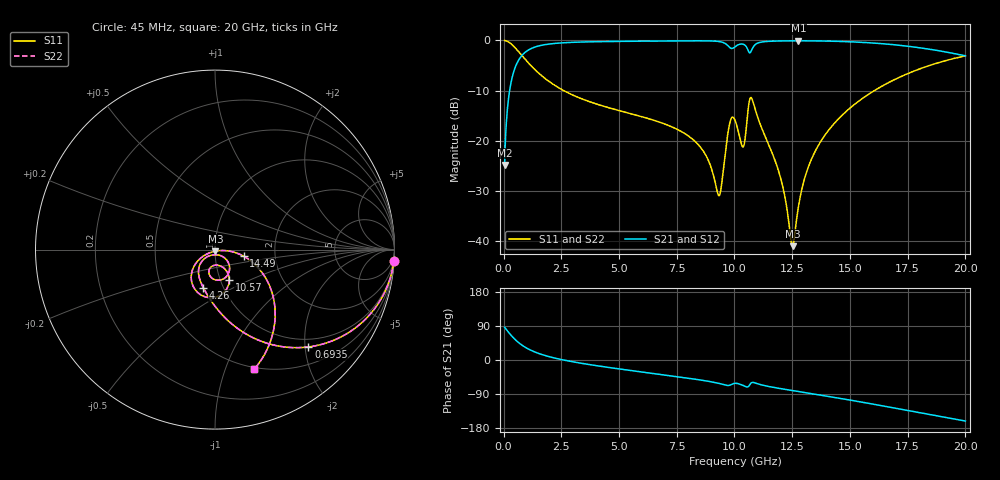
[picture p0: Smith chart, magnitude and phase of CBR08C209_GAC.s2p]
! S-parameter model data by Modelithics Inc.  support@modelithics.com 813-866-6335  Tampa FL USA
! S-Parameter data specifications:
! Substrate: 20-mil Rogers 4350B, substrate thickness, H=0.508mm, Dielectric constant, Er=3.75
! PCB Mounting Pad Footprint: Pad width, PadW=1.45mm , Pad length, PadL=1mm , Pad gap, PadG (edge-to-edge)=0.6mm , Reference planes=2.6mm apart
#  GHz  S  MA  R 50
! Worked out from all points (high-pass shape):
!   801 points, 45 MHz to 20 GHz, reference 50 ohm
!   highest |S21| = -0.09 dB at 12.77 GHz (marker M1); lowest = -24.8 dB at 45 MHz (marker M2)
!   |S21| within 3 dB of the highest: 779.9 MHz to end of sweep
!   lowest |S11| = -41.0 dB at 12.52 GHz (marker M3), VSWR 1.02, Z = 50.2 - j0.871 ohm
!   |S11| at or under -10 dB: 2.604 GHz to 16.06 GHz (13.46 GHz wide, 144 % of centre)
!   |S22| runs from -41.0 to 0.0 dB; largest |S21 - S12| = 0
!   S11 on the Smith chart (normalised r, x): 45 MHz: 1, -32; 693.5 MHz: 0.83, -2.07; 4.26 GHz: 0.81, -0.36; 10.57 GHz: 1.10, -0.38; 14.49 GHz: 1.38, -0.10; 20 GHz: 0.48, -1.26
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0.045  0.9983 -3.6  0.0573 86.4  0.0573 86.4  0.9983 -3.6
0.294438  0.9362 -22.7  0.3511 67.3  0.3511 67.3  0.9362 -22.7
0.693538  0.7514 -46.2  0.6591 43.7  0.6591 43.7  0.7514 -46.2
1.6414  0.4463 -75.1  0.8936 14.8  0.8936 14.8  0.4463 -75.1
3.387462  0.2616 -98.5  0.9634 -8.8  0.9634 -8.8  0.2616 -98.5
4.260494  0.2234 -106.7  0.9727 -17.1  0.9727 -17.1  0.2234 -106.7
6.704981  0.1547 -126.6  0.985 -37.4  0.985 -37.4  0.1547 -126.6
8.475988  0.08917 -139.0  0.9899 -52.3  0.9899 -52.3  0.08917 -139.0
9.324075  0.02834 -91.8  0.9744 -61.8  0.9744 -61.8  0.02834 -91.8
9.773062  0.1416 -55.4  0.8598 -66.8  0.8598 -66.8  0.1416 -55.4
10.0225  0.1601 -96.0  0.863 -61.5  0.863 -61.5  0.1601 -96.0
10.34677  0.08732 -91.5  0.9192 -66.5  0.9192 -66.5  0.08732 -91.5
10.57126  0.1856 -64.6  0.8142 -71.1  0.8142 -71.1  0.1856 -64.6
10.77081  0.257 -112.6  0.8246 -59.1  0.8246 -59.1  0.257 -112.6
11.76856  0.06243 -151.5  0.9844 -73.1  0.9844 -73.1  0.06243 -151.5
12.11777  0.03279 -148.5  0.9881 -76.7  0.9881 -76.7  0.03279 -148.5
12.51688  0.008916 -76.6  0.9899 -80.7  0.9899 -80.7  0.008916 -76.6
12.76631  0.02182 -15.8  0.9902 -83.2  0.9902 -83.2  0.02182 -15.8
13.36496  0.06807 -5.6  0.9887 -89.1  0.9887 -89.1  0.06807 -5.6
14.48743  0.1638 -13.0  0.9777 -100.4  0.9777 -100.4  0.1638 -13.0
16.68248  0.3808 -35.2  0.9151 -124.0  0.9151 -124.0  0.3808 -35.2
20  0.7013 -71.8  0.7017 -161.1  0.7017 -161.1  0.7013 -71.8
